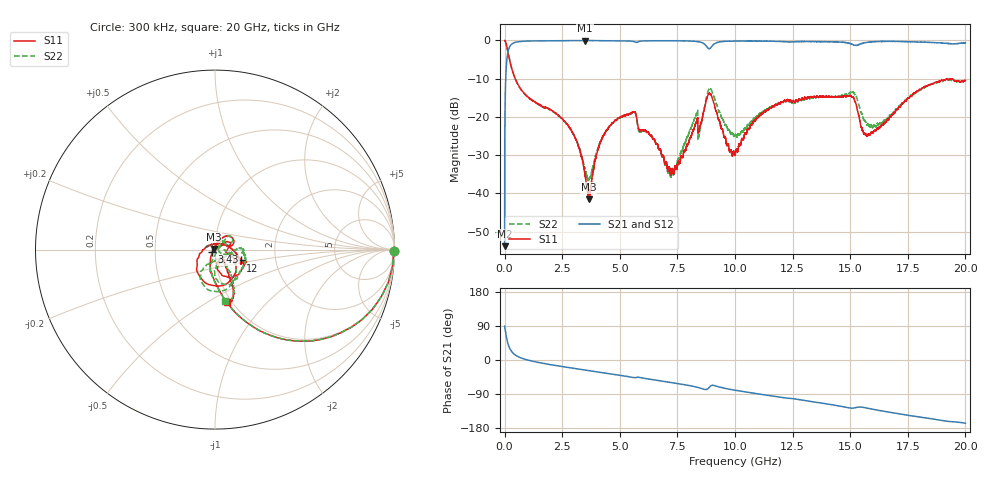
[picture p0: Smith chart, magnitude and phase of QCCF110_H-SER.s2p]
!{QCCF110}
!Johanson Technology Inc.
!www.johansontechnology.com
!Test Board Conditions:
!Substrate Type  RO4350B
!Substrate Thickness  10 mil
!Substrate Dk  3.66
!TL Type: GCPW
!TL Trace Width  21 mil
!TL Gap  20 mil
!Electrode orientation  Horizontal
!DUT TOPOLOGY	SERIES
!Mounting Pad LxW  16x21 mil
! Created Sat Jan  9 18:17:59 2021
# hz S ma R 50
! 2 Port Network Data from SP1.SP block
! freq  magS11  angS11  magS21  angS21  magS12  angS12  magS22  angS22
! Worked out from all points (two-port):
!   20001 points, 300 kHz to 20 GHz, reference 50 ohm
!   highest |S21| = -0.02 dB at 3.491 GHz (marker M1); lowest = -53.8 dB at 300 kHz (marker M2)
!   |S21| within 3 dB of the highest: 145 MHz to end of sweep
!   lowest |S11| = -41.6 dB at 3.652 GHz (marker M3), VSWR 1.02, Z = 49.2 + j0.327 ohm
!   |S11| at or under -10 dB: 461.5 MHz to 19.19 GHz (18.73 GHz wide, 191 % of centre); 19.19565 GHz to 19.19818 GHz (2.533 MHz wide, 0.0132 % of centre); 19.22 GHz to end of sweep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
!   |S22| runs from -36.6 to 0.0 dB; largest |S21 - S12| = 0.014
!   S11 on the Smith chart (normalised r, x): 300 kHz: open; 3.43 GHz: 0.97, -0.03; 12 GHz: 1.33, -0.16; 20 GHz: 0.95, -0.61
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300000  0.9964 -0.4  0.002043 89.4  0.002168 88.8  0.9953 -0.5
1.073e8  0.7997 -37.8  0.5968 51.9  0.5968 51.9  0.7995 -37.8
2.563e8  0.4937 -62.7  0.8636 26.7  0.8637 26.7  0.4933 -62.7
3.3343e9  0.03025 -128.8  0.9964 -25.1  0.9961 -25.0  0.03138 -91.9
3.4303e9  0.02236 -136.1  0.9959 -25.9  0.9961 -25.9  0.02481 -82.2
3.4913e9  0.01783 -143.6  0.9972 -26.5  0.9959 -26.5  0.0207 -75.7
3.6523e9  0.008359 156.6  0.9961 -28.0  0.9961 -28.0  0.01525 -30.8
4.1773e9  0.04817 68.9  0.9949 -32.8  0.9955 -32.8  0.04857 38.0
4.8643e9  0.09166 52.9  0.9916 -39.2  0.9905 -39.2  0.09092 45.7
5.6183e9  0.1169 30.6  0.9664 -46.5  0.9658 -46.6  0.1155 37.0
6.6673e9  0.04019 30.6  0.9905 -54.1  0.9904 -54.1  0.0405 50.1
7.2753e9  0.02026 64.1  0.9901 -59.7  0.989 -59.7  0.01976 -0.3
8.2863e9  0.08139 33.4  0.9711 -70.9  0.9702 -70.8  0.1012 -17.9
8.4873e9  0.07685 -16.2  0.9541 -74.1  0.9541 -74.0  0.06908 -13.1
8.9003e9  0.2026 -85.4  0.7811 -70.9  0.7779 -70.9  0.2343 -83.6
1.00003e10  0.03219 85.7  0.9836 -79.7  0.9827 -79.7  0.0584 -71.8
1.20003e10  0.1564 -22.8  0.9693 -98.6  0.9707 -98.5  0.1557 0.6
1.33343e10  0.1819 -22.5  0.9663 -109.7  0.9669 -109.7  0.1798 -17.3
1.50703e10  0.1819 -53.4  0.8971 -126.9  0.897 -127.4  0.211 -63.9
1.56813e10  0.05961 -57.5  0.9394 -126.4  0.9408 -126.4  0.08452 -77.4
1.66673e10  0.09215 -54.3  0.975 -137.2  0.9689 -137.8  0.1008 -55.3
2e10  0.2979 -77.3  0.9296 -166.9  0.9202 -166.8  0.2951 -78.6
